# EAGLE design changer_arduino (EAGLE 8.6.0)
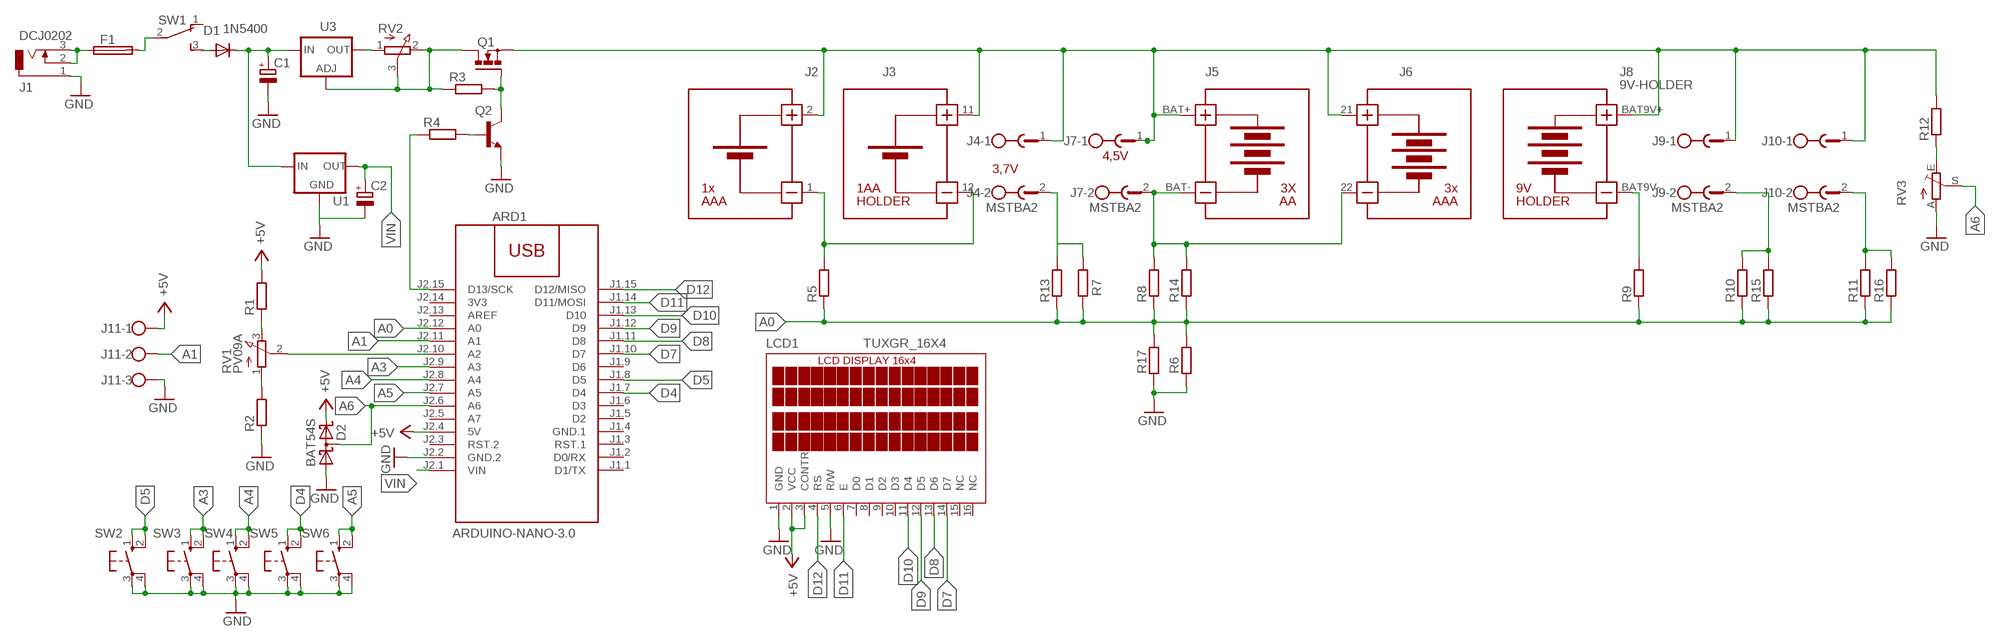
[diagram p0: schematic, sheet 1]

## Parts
ARD1  ARDUINO-NANO-3.0  [ARDUINO-NANO-3.0]
C1  CPOL-EUSMCD  [SMC_D]
C2  CPOL-EUSMCB  [SMC_B]
D1  1N5400  [DO201-15]
D2  BAT54S  [SOT23]
F1  FUSEGSH15  [GSH15]
J1  DCJ0202  [DCJ0202]
J2  BATTERY-HOLDER-1AAA  [BATTERY-HOLDER-1AAA]
J3  BATTERY-HOLDER-1AA  [BATTERY-HOLDER-1AA]
J4  MSTBA2  [MSTBA2]
J5  3AA  BATTERY-HOLDER-3AA  [BATTERY-HOLDER-3AA]
J6  BATTERY-HOLDER-3AAA  [BATTERY-HOLDER-3AAA]
J7  MSTBA2  [MSTBA2]
J8  9V-HOLDER  [9V-HOLDER]
J9  MSTBA2  [MSTBA2]
J10  MSTBA2  [MSTBA2]
J11  W237-103  [W237-103]
LCD1  TUXGR_16X4  [TUXGR_16X4]
Q1  BUZ11BV  [TO220BV]
Q2  BC337  [TO92]
R1  R-EU_R0805  [R0805]
R2  R-EU_R0805  [R0805]
R3  R-EU_R1206  [R1206]
R4  R-EU_R1206  [R1206]
R5  R-EU_R2512  [R2512]
R6  R-EU_R2512  [R2512]
R7  R-EU_R2512  [R2512]
R8  R-EU_R2512  [R2512]
R9  R-EU_R2512  [R2512]
R10  R-EU_R2512  [R2512]
R11  R-EU_R2512  [R2512]
R12  R-EU_R0805  [R0805]
R13  R-EU_R2512  [R2512]
R14  R-EU_R2512  [R2512]
R15  R-EU_R2512  [R2512]
R16  R-EU_R2512  [R2512]
R17  R-EU_R2512  [R2512]
RV1  PV09A  [PTV09]
RV2  POTPANEL  [POTPANELP231]
RV3  TRIM_EU-CA6V  [CA6V]
SW1  TL36YO  [TL3XYO]
SW2  40-XX  [B3F-40XX]
SW3  40-XX  [B3F-40XX]
SW4  40-XX  [B3F-40XX]
SW5  40-XX  [B3F-40XX]
SW6  40-XX  [B3F-40XX]
U1  78XXS  [78XXS]
U3  LM317MABT  [TO220L1]

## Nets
+5V: ARD1.J2.4(5V) D2.2(C2) J11.1 LCD1.2(VCC) LCD1.3(CONTR) R1.2
A0: ARD1.J2.12(A0) R5.1 R6.2 R7.1 R8.1 R9.1 R10.1 R11.1 R13.1 R14.1 R15.1 R16.1 R17.2
A1: ARD1.J2.11(A1) J11.2
A3: ARD1.J2.9(A3) SW3.1(S) SW3.2(S1)
A4: ARD1.J2.8(A4) SW4.1(S) SW4.2(S1)
A5: ARD1.J2.7(A5) SW6.1(S) SW6.2(S1)
A6: ARD1.J2.6(A6) D2.3(C1A2) RV3.S
D4: ARD1.J1.7(D4) SW5.1(S) SW5.2(S1)
D5: ARD1.J1.8(D5) SW2.1(S) SW2.2(S1)
D7: ARD1.J1.10(D7) LCD1.14(D7)
D8: ARD1.J1.11(D8) LCD1.13(D6)
D9: ARD1.J1.12(D9) LCD1.12(D5)
D10: ARD1.J1.13(D10) LCD1.11(D4)
D11: ARD1.J1.14(D11/MOSI) LCD1.6(E)
D12: ARD1.J1.15(D12/MISO) LCD1.4(RS)
GND: ARD1.J2.2(GND.2) C1.- C2.- D2.1(A1) J1.1 J11.3 LCD1.1(GND) LCD1.5(R/W) Q2.1(E) R2.1 R6.1 R17.1 RV3.A SW2.3(P) SW2.4(P1) SW3.3(P) SW3.4(P1) SW4.3(P) SW4.4(P1) SW5.3(P) SW5.4(P1) SW6.3(P) SW6.4(P1) U1.GND
N$1: F1.1 J1.2 J1.3
N$2: F1.2 SW1.2(P)
N$3: C1.+ D1.C U1.IN U3.3(IN)
N$4: D1.A SW1.3(S)
N$5: RV2.1(A) U3.2(OUT)
N$6: Q1.D R3.1 RV2.2(E) RV2.3(S) U3.1(ADJ)
N$7: Q1.G Q2.3(C) R3.2
N$8: Q2.2(B) R4.2
N$9: ARD1.J2.15(D13/SCK) R4.1
N$10: J2.1 J3.12 R5.2
N$11: J4.2 R7.2 R13.2
N$12: J5.BAT- J6.22(BAT-3XAAA-) J7.2 R8.2 R14.2
N$13: J8.BAT9V- R9.2
N$14: J2.2 J3.11 J4.1 J5.BAT+ J6.21(BAT3_3AAA+) J7.1 J8.BAT9V+ J9.1 J10.1 Q1.S R12.2
N$15: J10.2 R11.2 R16.2
N$16: J9.2 R10.2 R15.2
N$17: R1.1 RV1.3(E)
N$18: R2.2 RV1.1(A)
N$19: R12.1 RV3.E
N$20: ARD1.J2.10(A2) RV1.2(S)
VIN: ARD1.J2.1(VIN) C2.+ U1.OUT
Unconnected: ARD1.J1.1(D1/TX) ARD1.J1.2(D0/RX) ARD1.J1.3(RST.1) ARD1.J1.5(D2) ARD1.J1.6(D3) ARD1.J1.9(D6) ARD1.J2.3(RST.2) ARD1.J2.5(A7) ARD1.J2.13(AREF) LCD1.7(D0) LCD1.8(D1) LCD1.9(D2) LCD1.10(D3) LCD1.15(NC) LCD1.16(NC) SW1.1(O)

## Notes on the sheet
- 4,5V
- 3,7V

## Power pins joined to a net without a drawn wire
3V3: ARD1.J2.14(3V3)
GND.1: ARD1.J1.4(GND.1)

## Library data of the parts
ARD1 = diy-modules:ARDUINO-NANO-3.0: Arduino Nano 3.0 and compatible devices More details available here: https://www.arduino.cc/en/Main/ArduinoBoardNano Click here to find device on ebay.com
C1 C2 = rcl:CPOL-EU: POLARIZED CAPACITOR, European symbol
D1 = diode:1N5400: DIODE
D2 = diode:BAT54S: Schottky Diodes Pin connection corrected 2011-05-04 Source: Fairchild .. BAT54.pdf
F1 = fuse:FUSE: Fuse; OC_FARNELL: unknown; OC_NEWARK: unknown
J1 = con-jack:DCJ0202: DC POWER JACK Source: DCJ0202.pdf; OC_FARNELL: unknown; OC_NEWARK: unknown
J2 = diy-modules:BATTERY-HOLDER-1AAA
J3 = diy-modules:BATTERY-HOLDER-1AA
J4 J7 J9 J10 = con-phoenix-508:MSTBA2: PHOENIX; MF: FARNELL; MPN: 1757242; OC_FARNELL: 3705171; OC_NEWARK: 71C4161
J5 = diy-modules:BATTERY-HOLDER-3AA
J6 = diy-modules:BATTERY-HOLDER-3AAA
J8 = diy-modules:9V-HOLDER
J11 = con-wago-500:W237-103: WAGO SCREW CLAMP; MPN: 237-103; OC_FARNELL: unknown; OC_NEWARK: 18M7116
LCD1 = display-lcd:TUXGR_16X4
Q1 = transistor-power:BUZ11: N-CHANNEL MOS FET
Q2 = transistor:BC337: NPN TRANSISTOR
R1-R17 = rcl:R-EU_: RESISTOR, European symbol
RV1 = pot:PV09A
RV2 = pot:POTPANEL
RV3 = pot:TRIM_EU-: POTENTIOMETER
SW1 = switch:TL36YO: TINY SWITCH ON - ON Source: http://www2.produktinfo.conrad.com/datenblaetter/700000-724999/705152-da-01-de-Subminiaturschalter_TL_36YO.pdf
SW2-SW6 = switch-omron:40-XX: OMRON SWITCH; MF: OMRON COMPONENTS USA; MPN: B3F-4000; OC_FARNELL: 176434; OC_NEWARK: 36K3105
U1 = v-reg:78XXS: VOLTAGE REGULATOR
U3 = v-reg:LM317?*: 500 mA Adjustable Output Positive Voltage Regulator Source: http://www.onsemi.co.jp .. LM317M-D.PDF

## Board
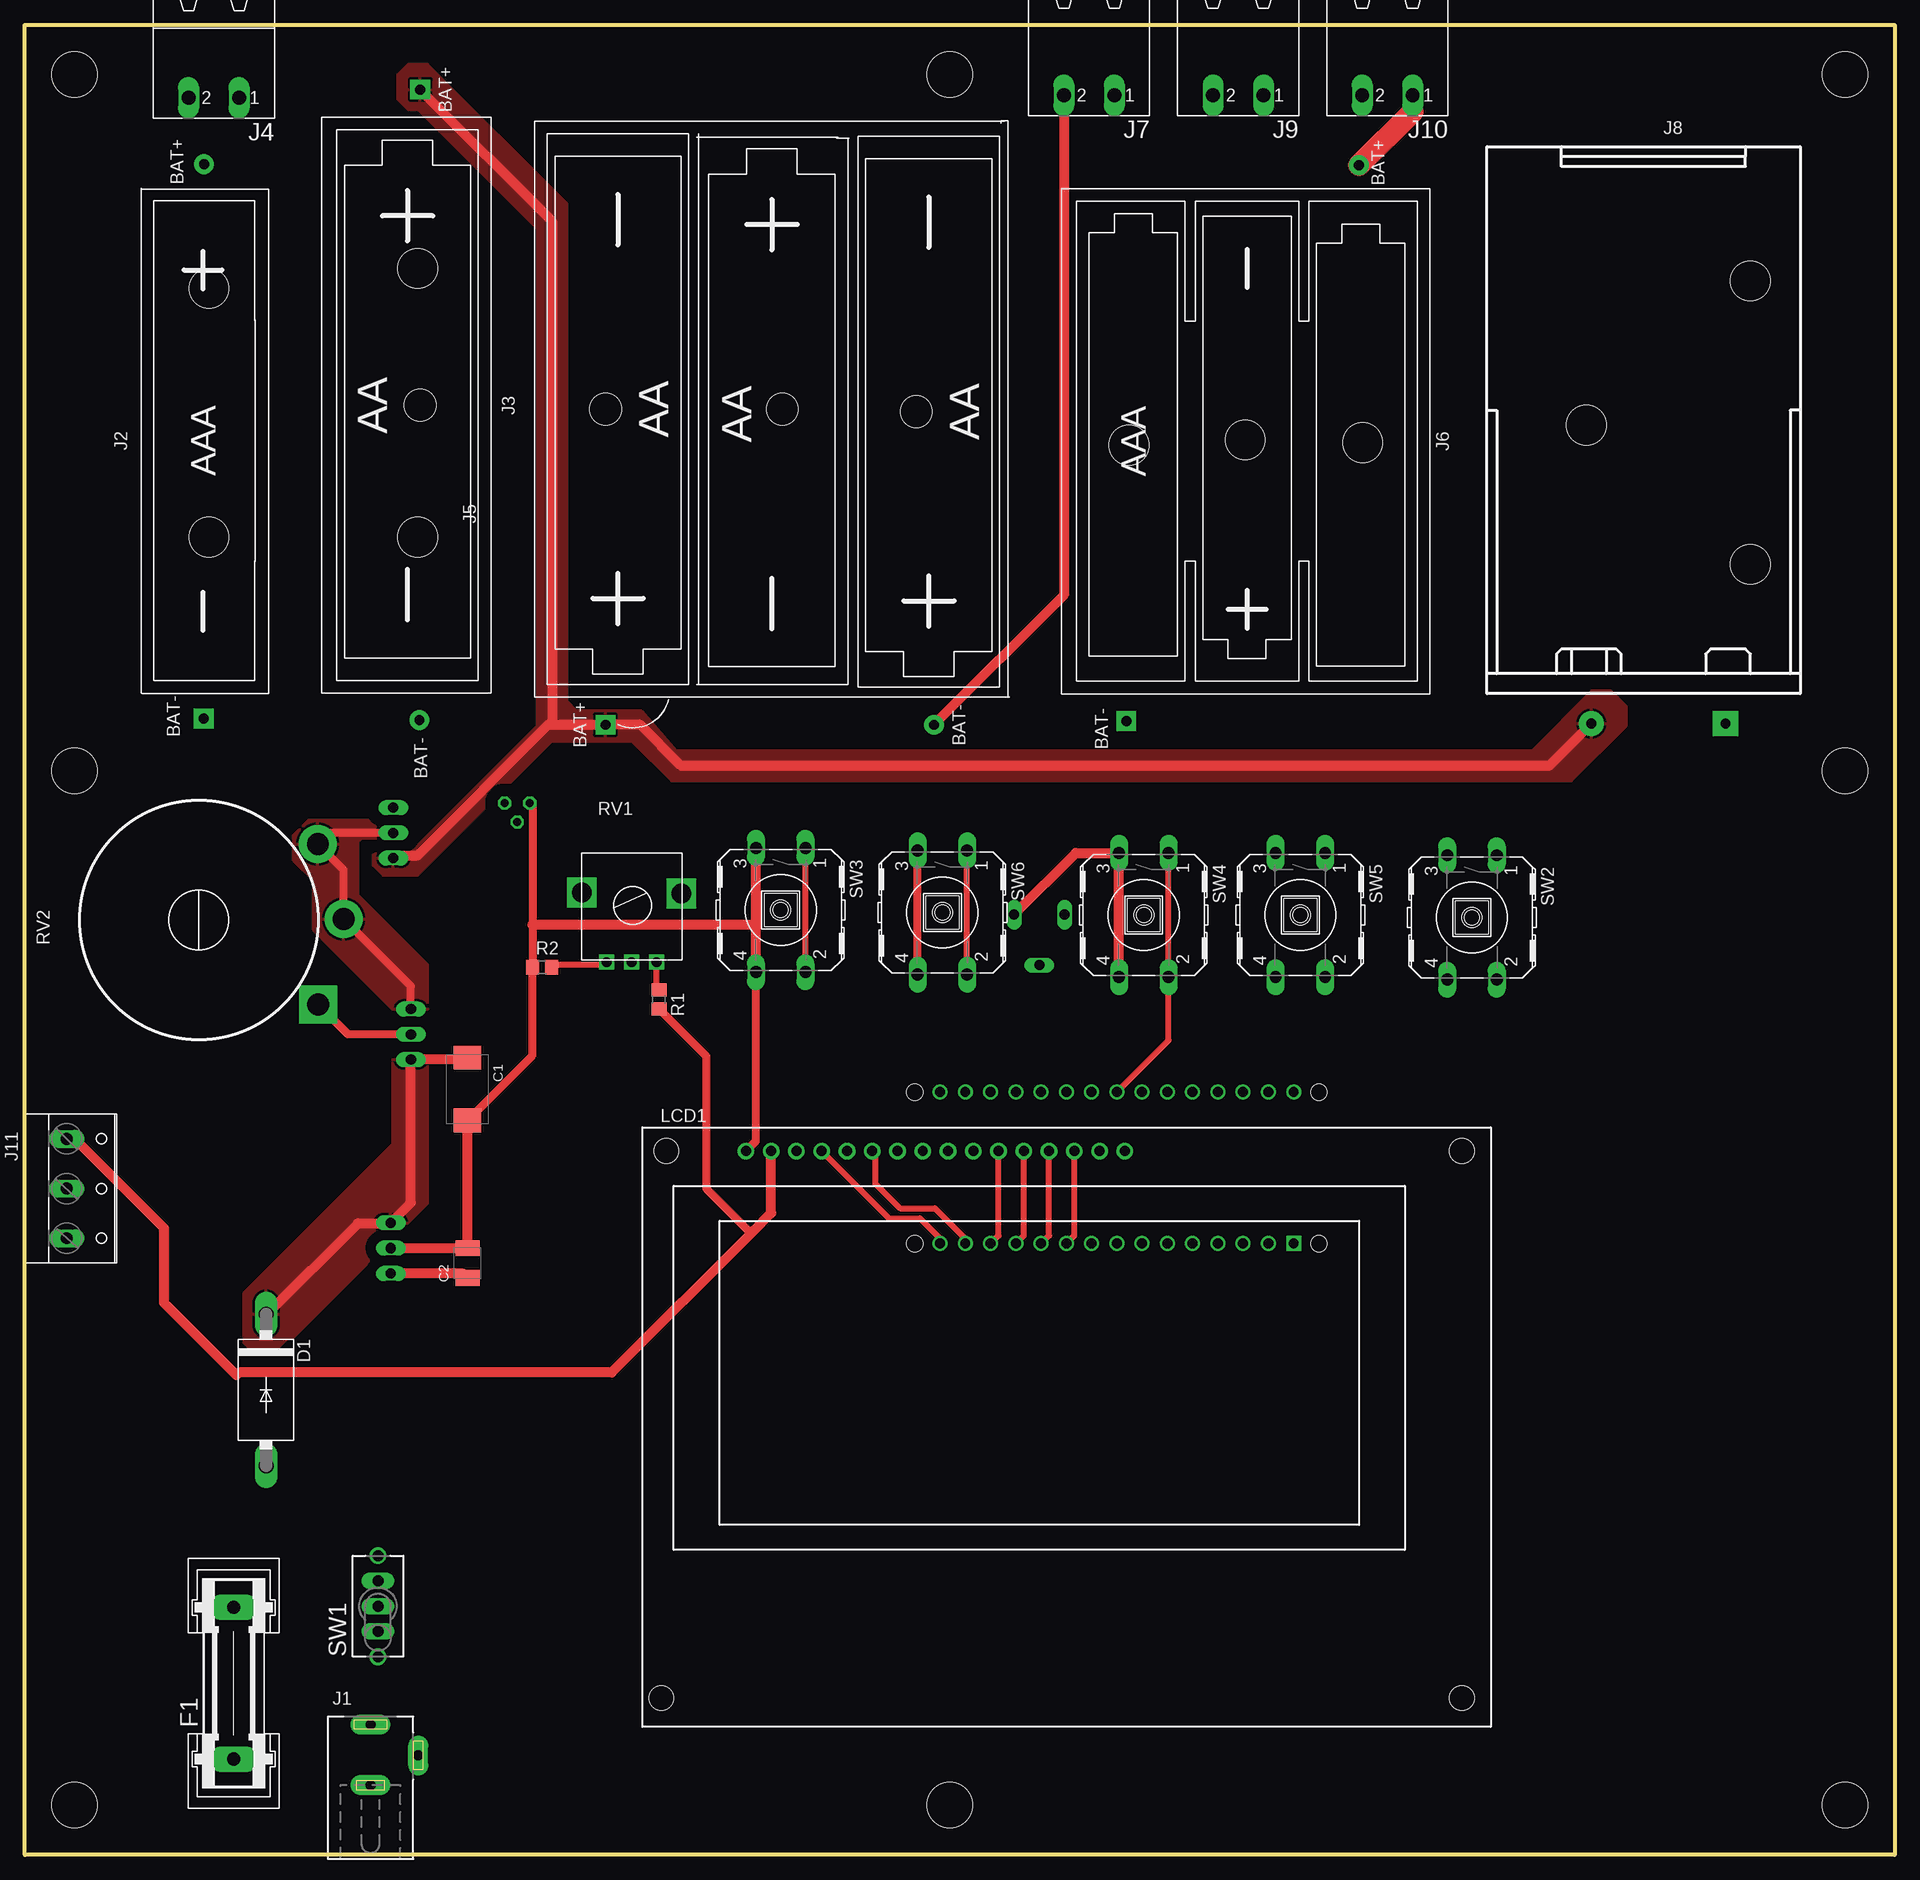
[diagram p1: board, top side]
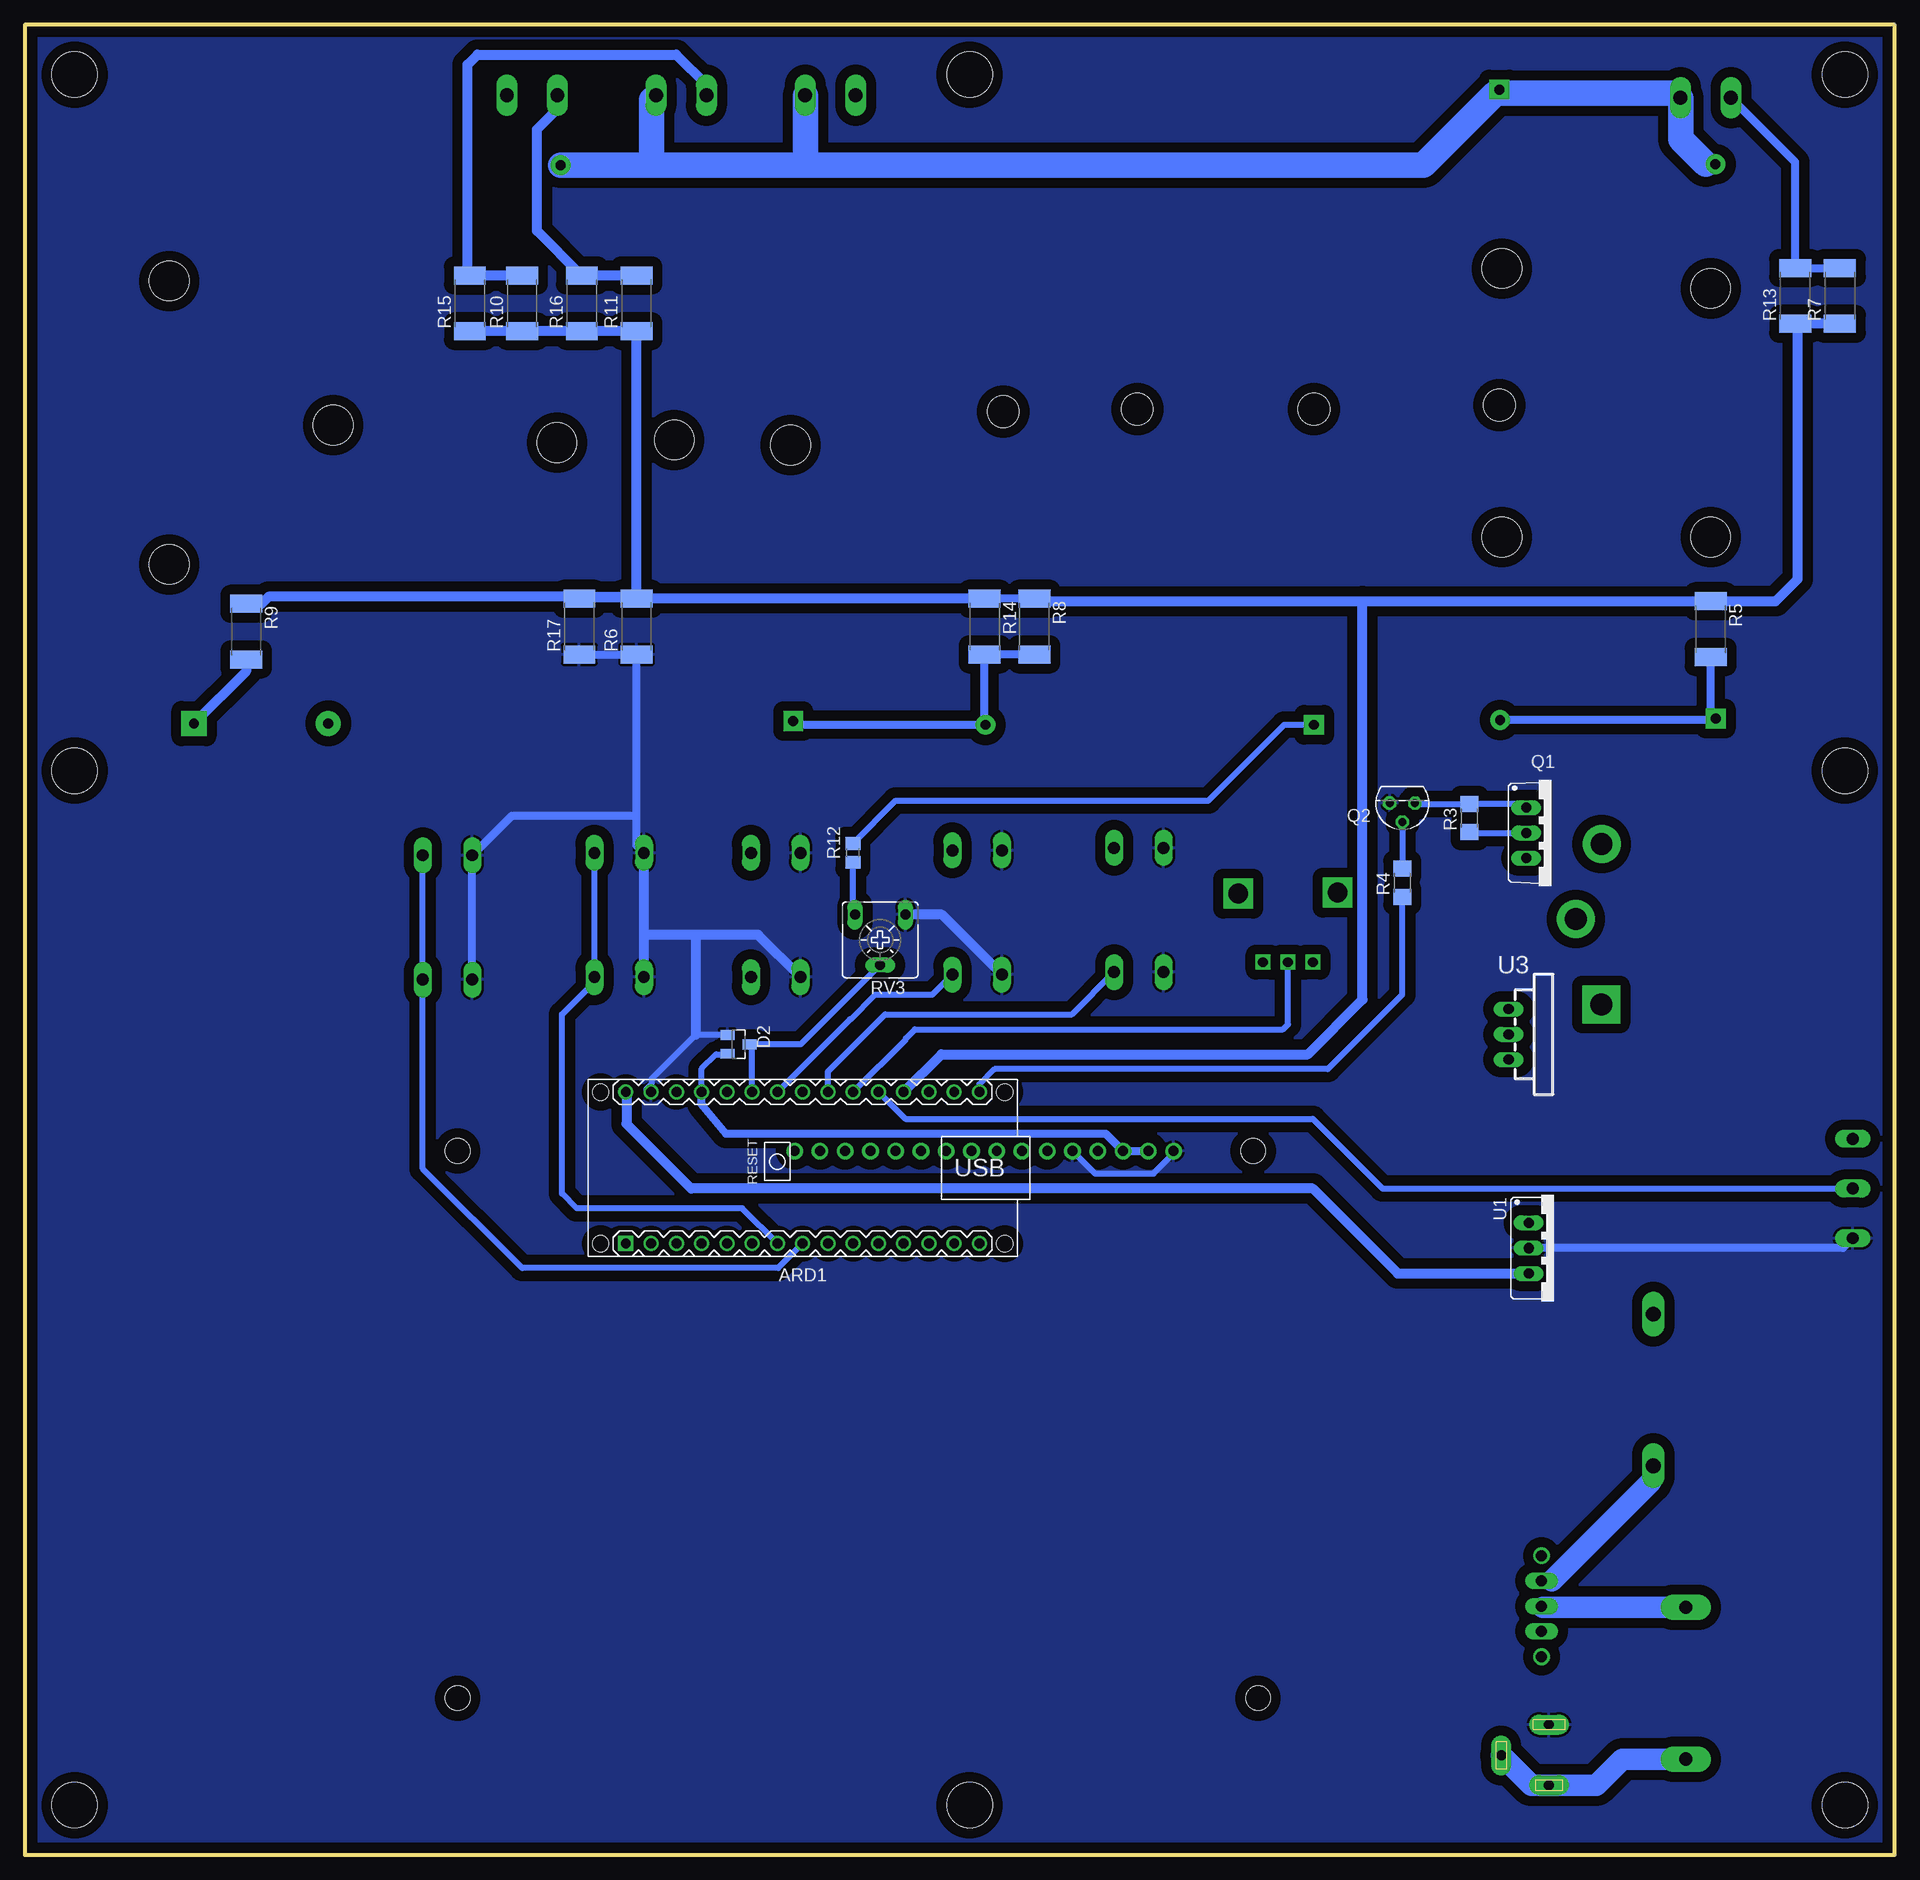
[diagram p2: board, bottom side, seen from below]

Size 188 x 184 mm. Coordinates in mm from the lower left corner, seen from the top.
Outline: 0,0 0,184 188,184 188,0 0,0
Copper layers (1*16): Top 0.035mm / dielectric 1.5mm / Bottom 0.035mm
Design rules "default": minimum track width 10mil, minimum drill 24mil, track to track 8mil, track to pad 8mil, pad to pad 8mil, via to via 8mil, smd to smd 8mil, copper to edge 40mil, drill to drill 8mil, minimum pad ring 10mil, minimum via ring 8mil, stop-mask expansion 4mil, vias tented up to drill 0mil, thermal gap 10mil
Holes 4.6 mm at 5,5 93,5 183,5 5,109 183,109 5,179 93,179 183,179
Holes 4 mm at 18.5,132.5 18.5,157.5 39.5,132.5 39.5,159.5

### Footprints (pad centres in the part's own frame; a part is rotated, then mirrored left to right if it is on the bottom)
ARDUINO-NANO-3.0 = drill 1 square: J1.1 17.78,7.62 | drill 1: J1.2 15.24,7.62; J1.3 12.7,7.62; J1.4 10.16,7.62; J1.5 7.62,7.62; J1.6 5.08,7.62; J1.7 2.54,7.62; J1.8 0,7.62; J1.9 -2.54,7.62; J1.10 -5.08,7.62; J1.11 -7.62,7.62; J1.12 -10.16,7.62; J1.13 -12.7,7.62; J1.14 -15.24,7.62; J1.15 -17.78,7.62; J2.1 17.78,-7.62; J2.2 15.24,-7.62; J2.3 12.7,-7.62; J2.4 10.16,-7.62; J2.5 7.62,-7.62; J2.6 5.08,-7.62; J2.7 2.54,-7.62; J2.8 0,-7.62; J2.9 -2.54,-7.62; J2.10 -5.08,-7.62; J2.11 -7.62,-7.62; J2.12 -10.16,-7.62; J2.13 -12.7,-7.62; J2.14 -15.24,-7.62; J2.15 -17.78,-7.62 | hole 1.651: -20.32,7.62; -20.32,-7.62; 20.32,-7.62; 20.32,7.62
SMC_D = smd 2.4 x 2.8: + -3.15,0; - 3.15,0
SMC_B = smd 1.6 x 2.4: + -1.5,0; - 1.5,0
DO201-15 = drill 1.499 long: A 7.62,0; C -7.62,0
SOT23 = smd 1 x 1.4: 1 -0.95,-1.1; 2 0.95,-1.1; 3 0,1.1
GSH15 = drill 1.321 pad 2.54 long: 1 -7.62,0; 2 7.62,0
DCJ0202 = drill 1 pad 2 long: 1 0,3.1; 2 4.8,0; 3 0,-3
BATTERY-HOLDER-1AAA = drill 1 pad 2 square: 1 0,0 | drill 1 pad 2: 2 55.75,-0.01
BATTERY-HOLDER-1AA = drill 1 pad 2 square: 11 0,0 | drill 1 pad 2: 12 63.4,-0.08 | hole 3.2: 31.75,0
MSTBA2 = drill 1.397 long: 1 -2.54,5.08; 2 2.54,5.08
BATTERY-HOLDER-3AA = drill 1 pad 2 square: BAT+ 0,0 | drill 1 pad 2: BAT- 0,-33.03 | hole 3.2: 31.75,0; 31.75,-17.78; 31.5,-31.25
BATTERY-HOLDER-3AAA = drill 1 pad 2: 21 -28.375,11.89 | drill 1 pad 2 square: 22 27.505,-11.51 | hole 4: -0.5,12.25; -0.25,-11.25; -0.77,0.45
9V-HOLDER = drill 1 pad 2.54: BAT9V+ 58,-21 | drill 1 pad 2.54 square: BAT9V- 58,-7.5 | hole 4: 13.5,-5; 42,-5; 28,-21.5
W237-103 = drill 1.194 long: 1 -5,-1.29; 2 0,-1.29; 3 5,-1.29
TUXGR_16X4 = drill 1 pad 1.676: 1 2.25,0.26; 2 4.79,0.26; 3 7.33,0.26; 4 9.87,0.26; 5 12.41,0.26; 6 14.95,0.26; 7 17.49,0.26; 8 20.03,0.26; 9 22.57,0.26; 10 25.11,0.26; 11 27.65,0.26; 12 30.19,0.26; 13 32.73,0.26; 14 35.27,0.26; 15 37.81,0.26; 16 40.35,0.26 | hole 2.5: -6.25,-54.74; 74.25,-54.74; -5.75,0.26; 74.25,0.26
TO220BV = drill 1.016 long: D 0,-2.54; G -2.54,-2.54; S 2.54,-2.54
TO92 = drill 0.813 octagon: 1 1.27,0; 2 0,1.905; 3 -1.27,0
R0805 = smd 1.3 x 1.5: 1 -0.95,0; 2 0.95,0
R1206 = smd 1.6 x 1.803: 1 -1.422,0; 2 1.422,0
R2512 = smd 1.8 x 3.2: 1 -2.8,0; 2 2.8,0
PTV09 = drill 1 square: 1 -2.5,0; 2 0,0; 3 2.5,0 | drill 2 square: P$4 -5,7; P$5 5,6.9
POTPANELP231 = drill 2.2 pad 3.81 square: 1 -8.5,-12 | drill 2.2 pad 3.81: 2 7.62,-11.96; 3 0.11,-14.54
CA6V = drill 1.016 long: A -2.54,-2.54; E 2.54,-2.54; S 0,2.54
TL3XYO = drill 1.1 pad 1.422 long: 1 -2.54,0; 2 0,0; 3 2.54,0 | drill 1.1 pad 1.676: M1 -5.08,0; M2 5.08,0
B3F-40XX = drill 1.194 long: 1 -6.248,2.489; 2 6.248,2.489; 3 -6.248,-2.489; 4 6.248,-2.489
78XXS = drill 1.016 long: GND 0,-2.54; IN -2.54,-2.54; OUT 2.54,-2.54
TO220L1 = drill 1.016 long: 1 -2.54,-3.81; 2 0,-3.81; 3 2.54,-3.81

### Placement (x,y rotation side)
ARD1  109.8,69.08 180 bottom
C1  44.5,77 270 top
C2  44.5,59.5 90 top
D1  24.25,46.75 270 top
D2  116.25,81.5 270 bottom
F1  21,17.25 90 top
J1  34.75,10 0 top
J2  18,114.25 90 top
J3  39.75,177.5 270 top
J4  19,181.75 180 top
J5  58.38,113.62 90 top
J6  122.25,141.5 270 top
J7  107,182 180 top
J8  178.5,171.75 270 top
J9  122,182 180 top
J10  137,182 180 top
J11  5.5,67 270 top
LCD1  70.25,70.5 0 top
Q1  34.5,102.75 270 bottom
Q2  49.5,105.75 180 bottom
R1  63.75,86 270 top
R2  52,89.25 0 top
R3  42.75,104.25 90 bottom
R4  49.5,97.75 90 bottom
R5  18.5,123.25 270 bottom
R6  126.5,123.5 90 bottom
R7  5.5,156.75 90 bottom
R8  86.5,123.5 270 bottom
R9  165.75,123 270 bottom
R10  138,156 90 bottom
R11  126.5,156 90 bottom
R12  104.75,100.75 90 bottom
R13  10,156.75 90 bottom
R14  91.5,123.5 270 bottom
R15  143.25,156 90 bottom
R16  132,156 90 bottom
R17  132.25,123.5 90 bottom
RV1  61,89.75 0 top
RV2  17.5,94 90 top
RV3  102,92 180 bottom
SW1  35.5,25 90 top
SW2  145.5,94.25 270 top
SW3  76,95 270 top
SW4  112.5,94.5 270 top
SW5  128.25,94.5 270 top
SW6  92.25,94.75 270 top
U1  34.25,61 270 bottom
U3  35,82.5 270 bottom

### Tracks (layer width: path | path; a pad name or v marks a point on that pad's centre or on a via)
+5V
  Top 0.813: R1.2 68.5,80.3 68.5,67 72.75,62.75 73.25,62.75
  Top 1.016: J11.1 5,72 14,63 14,55.5 21.25,48.25 21.5,48.5 59,48.5 73.25,62.75 75.04,64.54 LCD1.2
  Bottom 0.61: ARD1.J2.4 119.95,79.05 118.5,80.5 117.4,80.5 D2.2
  Bottom 0.813: LCD1.2 LCD1.3 79.32,72.5 117.5,72.5 119.95,75.45 ARD1.J2.4
A0
  Bottom 0.61: 18,126 18.05,126.05 R5.1
  Bottom 0.813: 86.25,126.05 R8.1 R14.1 | R6.2 R17.2
  Bottom 1: 86.25,126.05 53.5,126.05 R5.1 | R14.1 R6.2
  Bottom 1.016: R15.1 R10.1 R16.1 R11.1 126.5,126.5 132.05,126.5 R17.2 132.45,126.5 163.5,126.5 164.2,125.8 R9.1 | ARD1.J2.12 95.83,80.5 59,80.5 53.5,86 53.5,126.05 | 18.05,126.05 11.95,126.05 9.75,128.25 9.75,153.7 R13.1 R7.1
A1
  Bottom 0.61: ARD1.J2.11 99.47,74 58.5,74 51.5,67 J11.2
A3
  Top 0.61: SW3.2 SW3.1
  Bottom 0.61: ARD1.J2.9 107.25,78.75 101.5,84.5 82.74,84.5 SW3.2
A4
  Top 0.61: ARD1.J2.8 114.99,81.89 SW4.2 SW4.1
A5
  Top 0.61: SW6.2 SW6.1
  Bottom 0.61: ARD1.J2.7 105.03,84 105,84 102.5,86.5 96.74,86.5 SW6.2
A6
  Bottom 0.61: RV3.S 102.04,89.46 110,81.5 D2.3 114.88,81.22 ARD1.J2.6
D4
  Bottom 0.61: ARD1.J1.7 115.88,65 132.5,65 134,66.5 134,84.5 130.74,87.76 SW5.2 SW5.1
D5
  Bottom 0.61: ARD1.J1.8 112.25,59 138,59 147.99,68.99 SW2.2 SW2.1
D7
  Top 0.61: ARD1.J1.10 105.52,62.27 LCD1.14
D8
  Top 0.61: ARD1.J1.11 102.98,62.27 LCD1.13
D9
  Top 0.61: ARD1.J1.12 100.44,62.27 LCD1.12
D10
  Top 0.61: ARD1.J1.13 97.9,62.27 LCD1.11
D11
  Top 0.61: LCD1.6 85.5,70.46 85.5,67.5 88,65 91.5,65 94.56,61.95 ARD1.J1.14
D12
  Top 0.61: LCD1.4 86.88,64 90,64 92.02,61.98 ARD1.J1.15
GND
  Top 0.813: LCD1.1 73.51,71.77 SW3.4 | C1.- 51.05,80.4 R2.1 51.05,93.5 51.05,105.47 Q2.1 | SW6.4 SW6.3
  Top 1.016: C1.- C2.- U1.GND | SW3.3 SW3.4 73.5,88.76 73.5,93.5 51.05,93.5 | RV3.A 105.67,100.75 SW4.3 SW4.4
  Bottom 0.61: D2.1 120.55,82.45 125,78 125,77.5 125.5,77 ARD1.J2.2 | LCD1.5 80.4,68.5 74.5,68.5 72.5,70.5 LCD1.1
  Bottom 0.813: R17.1 R6.1 126.5,104.5 | SW5.3 126.5,101.49 126.5,104.5 | J11.3 5.21,61 U1.GND | SW2.4 SW2.3 139.01,104.5 126.5,104.5
  Bottom 1.016: SW6.4 95.8,94.54 RV3.A | SW5.4 125.76,92.5 | 125.76,92.5 SW5.3 | SW4.4 114.26,92.5 120.5,92.5 | 120.5,92.5 125.76,92.5 | 120.55,82.45 120.5,82.5 120.5,92.5
  pour Bottom (isolate 1.016): 0.5,183.5 187,183.5 187,0.5 0.5,0.5
N$1
  Bottom 2.184: F1.1 27.37,9.63 30,7 J1.3 36.55,7 J1.2
N$2
  Bottom 1.016: 35.37,24.87 SW1.2
  Bottom 2.184: F1.2 35.37,24.87
N$3
  Top 1.016: C1.+ 44.31,79.96 U3.3 38.81,65.56 U1.IN 36.75,63.5 33.5,63.5 24.37,54.37 D1.C
  pour Top (isolate 1.016): 37,80.5 37,71.5 22,56.5 22,51.5 22.5,51 25.5,51 26.5,52 27,52 40.5,65.5 40.5,80.5 40,81 37.5,81
N$4
  Bottom 1.016: SW1.3 34.46,27.54 | 24.5,37.5 24.5,38.88 D1.A
  Bottom 2.184: 34.46,27.54 24.5,37.5
N$5
  Top 0.813: U3.2 32.5,82.5 RV2.1
N$6
  Top 0.813: Q1.D 30.59,102.75 RV2.2 32.04,99.04 RV2.3 38.81,87.34 U3.1
  Bottom 0.61: R3.1 42.67,102.75 Q1.D
  pour Top (isolate 1.27, rank 2): 38,84 39.5,84 40.5,85 40.5,89.5 33.5,96.5 33.5,100.5 34.5,101.5 38.5,101.5 39,102 39,104 28.5,104 27,102.5 27,100 29,98 29,93
N$7
  Bottom 0.61: Q2.3 48.15,105.67 R3.2 37.42,105.67 Q1.G
N$8
  Bottom 0.61: Q2.2 R4.2
N$9
  Bottom 0.61: R4.1 49.5,86.5 57,79 90.5,79 92.02,77.48 ARD1.J2.15
N$10
  Bottom 0.813: R5.2 18.5,114.75 J2.1 18.15,114.1 J3.12
N$11
  Bottom 0.813: J4.2 10,170.21 R13.2 R7.2
N$12
  Top 1.016: J7.2 104.46,126.68 J5.BAT-
  Bottom 0.813: R8.2 R14.2 91.5,113.72 J5.BAT- 110.37,113.62 J6.22
N$13
  Bottom 1.016: R9.2 165.75,119 J8.BAT9V-
N$14
  Top 1.016: Q1.S 37.33,100.5 39.5,100.5 52.62,113.62 53,113.62 | 53,113.62 57,113.62 J5.BAT+ 61.88,113.62 66,109.5 153.25,109.5 J8.BAT9V+ | 139.54,175.28 J10.1 | J3.11 53,164.25 53,113.62
  Top 2.184: J6.21 139.54,175.28
  Bottom 0.61: R12.2 100.45,106 69,106 61.38,113.62 J5.BAT+
  Bottom 1.016: J7.1 109.5,176.88 | J9.1 125,176.46 | 40.12,177.12 J3.11 | 22,177.12 J4.1 21.5,176.63 | 19,170 J2.2
  Bottom 2.54: 109.5,169.88 47.38,169.88 40.12,177.12 22,177.12 | 109.5,169.88 125,169.88 | 125,169.88 J6.21 | 109.5,176.88 109.5,169.88 | 125,176.46 125,169.88 | 21.5,176.63 21.5,172.5 19,170
  pour Top (isolate 1.27): 36,101.5 35,100.5 35,99.5 36,98.5 39.5,98.5 53,112 61,112 65,108 155.5,108 161,113.5 161,115.5 159.5,117 157.5,117 151.5,111 65.5,111 62,115 55.5,115 54.5,116 54.5,166 40.5,180 38.5,180 37.5,179 37.5,176.5 38.5,175.5 39.5,175.5 51.5,163.5 51.5,113.5 39,101
N$15
  Bottom 1.016: J10.2 134.46,175.54 136.5,173.5 136.5,163.3 R16.2 R11.2
N$16
  Bottom 1.016: J9.2 119.46,177.96 122.5,181 142.5,181 143.5,180 143.5,159.05 R15.2 R10.2
N$17
  Top 0.61: R1.1 63.5,87.2 RV1.3
N$18
  Top 0.61: R2.2 53.2,89.5 58,89.5 58.25,89.75 RV1.1
N$19
  Bottom 0.61: RV3.E 104.75,94.75 R12.1
N$20
  Bottom 0.61: ARD1.J2.10 99.42,82 99.42,82.08 98.5,83 61.5,83 61,83.5 RV1.2
VIN
  Top 1.016: C2.+ 44.04,58.46 U1.OUT
  Bottom 1.016: ARD1.J2.1 127.5,76.62 127.5,73.5 121,67 58.5,67 49.96,58.46 U1.OUT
